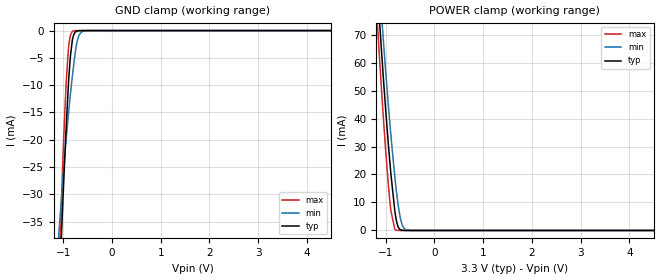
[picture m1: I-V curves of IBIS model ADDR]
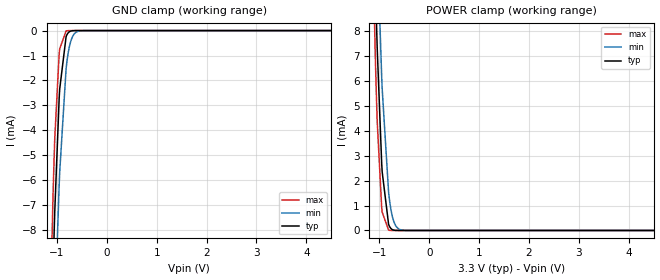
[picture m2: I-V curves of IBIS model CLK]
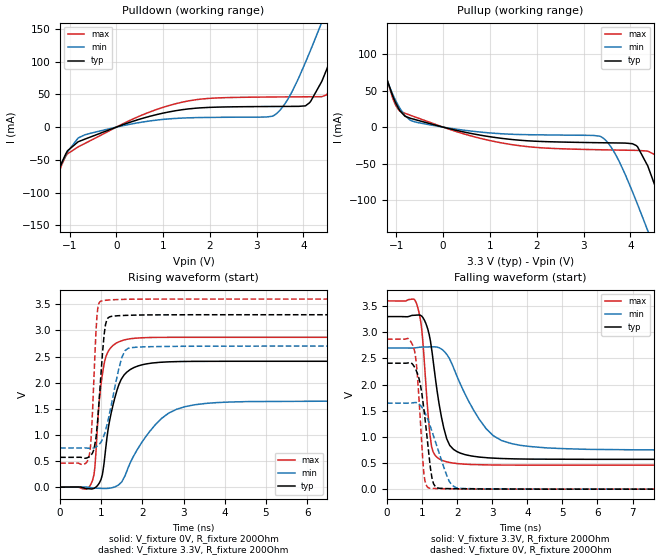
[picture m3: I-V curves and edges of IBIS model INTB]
|Texas Instruments Incorporated
| Marketing part#   Digital Voltage Range   Package-type   #pins
| FDC2114   2.7V-3.6V   QFN   16
[IBIS Ver]   4.1
[File name]   fdc2114.ibs
[File Rev]   1.0
[Date]   12/10/2014
[Source]
| Texas Instruments Incorporated.
| 12500 TI Blvd
| Dallas, TX -75243
[Notes]   Revision History:
| Rev 1.0: 12/10/2014
| - Initial version of the model
| - Model generated from simulations in TISPICE
| - C_comp although listed in numerical order of value are
|   obtained from varying PVT conditions. For PVT conditions for
|   each specific value refer the buffer description under
|   respective [Model]. IBIS model user is responsible for using
|   appropriate C_comp to simulate for Signal Integrity.
| - Warnings regarding combined Non-monotonicity of various models have been
|   reviewd and considered minor and can be ignored.
[Disclaimer]
| This model is designed as an aid for customers of Texas Instruments.
| TI and its licensors and suppliers make no warranties, either expressed
| or implied, with respect to this  model, including the warranties of
| merchantability or fitness for a particular purpose. The model is
| provided solely on an "as is" basis. The entire risk as to its quality
| and performance is with the customer.
[Copyright]
 (C) Copyright 2014 Texas Instruments Incorporated.All rights reserved.
|   Device
[Component]   FDC2114
[Manufacturer]   TI
[Package]
| QFN   16
|   typ   min   max
R_pkg   0.055   0.033   0.082
L_pkg   0.881nH   0.624nH   1.131nH
C_pkg   0.218pF   0.183pF   0.252pF
[Pin]  signal_name   model_name   R_pin   L_pin   C_pin
1   SCL   SCL   0.07306   0.978nH   0.18274pF
2   SDA   SDA   0.07559   1.01766nH   0.20668pF
3   CKIN   CLK   0.07543   1.01504nH   0.20688pF
4   ADDR   ADDR   0.08092   1.10425nH   0.19068pF
5   INTB   INTB   0.08236   1.13165nH   0.19465pF
6   SD   ADDR   0.08179   1.12348nH   0.21458pF
7   VDD   POWER   0.07866   1.06968nH   0.21147pF
8   GND   GND   0.04053   0.79295nH   0.22494pF
9   IN0A   NC   0.04363   0.92929nH   0.23597pF
10   IN0B   NC   0.03905   0.78694nH   0.25179pF
11   IN1A   NC   0.03767   0.74474nH   0.2462pF
12   IN1B   NC   0.03662   0.71322nH   0.21859pF
13   IN2A   NC   0.03341   0.62974nH   0.20896pF
14   IN2B   NC   0.03331   0.62362nH   0.23291pF
15   IN3A   NC   0.03436   0.6538nH   0.23712pF
16   IN3B   NC   0.03859   0.786nH   0.22133pF
| Models and submodels in the file (5): ADDR (Input), CLK (Input), INTB (Output), SCL (Input), SDA (I/O_open_drain)
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|   Model
[Model]   ADDR
Model_type   Input
Vinl = 0.99
Vinh = 2.31
|   typ   min   max
C_comp   0.676pF   0.666pF   0.695pF
[Voltage Range]   3.3   2.7   3.6
[Temperature Range]   27   125   -40
[Power Clamp Reference]   3.3   2.7   3.6
[GND Clamp Reference]   0   0   0
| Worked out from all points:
|   GND clamp passes 1 mA (typ) near -0.79 V on its own axis
|   POWER clamp passes 1 mA (typ) near -0.74 V on its own axis
[GND Clamp]
|   Voltage   I(typ)   I(min)   I(max)
-3.3V     -619.4mA   -393.3mA   -763.1mA
-1.092V   -49.22mA   -37.35mA   -44.76mA
-1.003V   -30.19mA   -26.61mA   -22.47mA
-943.8mV  -18.39mA   -20.21mA   -10.3mA
-894.3mV  -9.845mA   -15.28mA   -3.327mA
-854.7mV  -4.809mA   -11.73mA   -852.6uA
-815.1mV  -1.831mA   -8.493mA   -184uA
-795.3mV  -1.044mA   -6.986mA   -84.86uA
-735.9mV  -170.8uA   -2.934mA   -6.707uA
-696.3mV  -49.54uA   -1.348mA   -1.028uA
-547.8mV  -263.7nA   -41.3uA    0A
6.6V      0A         0A         0A
[POWER Clamp]
|   Voltage   I(typ)   I(min)   I(max)
-3.3V     741.9mA    707.9mA    777.5mA
-1.211V   97.25mA    108.2mA    85.62mA
-1.142V   78.32mA    90.49mA    65.34mA
-1.092V   65.31mA    78.23mA    51.56mA
-1.053V   55.31mA    68.69mA    41.1mA
-943.8mV  30.12mA    44.08mA    15.79mA
-894.3mV  20.1mA     33.88mA    6.969mA
-815.1mV  7.134mA    19.29mA    506.1uA
-785.4mV  3.858mA    14.56mA    134.6uA
-676.5mV  121.2uA    2.795mA    1.023uA
-528mV    587.8nA    67.21uA    0A
6.6V      0A         0A         0A
|   Model
[Model]   CLK
Model_type   Input
Vinl = 0.99
Vinh = 2.31
|   typ   min   max
C_comp   0.594pF   0.592pF   0.599pF
[Voltage Range]   3.3   2.7   3.6
[Temperature Range]   27   125   -40
[Power Clamp Reference]   3.3   2.7   3.6
[GND Clamp Reference]   0   0   0
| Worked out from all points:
|   GND clamp passes 1 mA (typ) near -0.86 V on its own axis
|   POWER clamp passes 1 mA (typ) near -0.86 V on its own axis
[GND Clamp]
|   Voltage   I(typ)   I(min)   I(max)
-3.3V     -281.2mA   -260.7mA   -298mA
-1.162V   -16.92mA   -20.78mA   -14.06mA
-1.082V   -10.12mA   -14.36mA   -7.027mA
-1.063V   -8.64mA    -12.89mA   -5.599mA
-1.053V   -7.94mA    -12.19mA   -4.947mA
-1.043V   -7.269mA   -11.49mA   -4.339mA
-953.7mV  -2.688mA   -6.162mA   -914.3uA
-815.1mV  -242.9uA   -1.528mA   -13.45uA
-765.6mV  -74.11uA   -807.8uA   -1.597uA
-706.2mV  -13.3uA    -337.5uA   -98.92nA
-518.1mV  -14.83nA   -7.449uA   0A
6.6V      0A         0A         0A
[POWER Clamp]
|   Voltage   I(typ)   I(min)   I(max)
-3.3V     281.2mA    260.7mA    298mA
-1.162V   16.92mA    20.78mA    14.06mA
-1.082V   10.12mA    14.36mA    7.027mA
-1.063V   8.64mA     12.89mA    5.599mA
-1.053V   7.94mA     12.19mA    4.947mA
-1.043V   7.269mA    11.49mA    4.339mA
-953.7mV  2.688mA    6.162mA    914.3uA
-815.1mV  242.9uA    1.528mA    13.45uA
-765.6mV  74.11uA    807.8uA    1.597uA
-706.2mV  13.3uA     337.5uA    99.01nA
-518.1mV  15.01nA    7.449uA    0A
6.6V      0A         0A         0A
|   Model
[Model]   INTB
Model_type   Output
Polarity   Non-Inverting
Vmeas = 1.65
Vref = 0
Cref = 1pF
Rref = 100000
|   typ   min   max
C_comp   0.767pF   0.749pF   0.775pF
[Voltage Range]   3.3   2.7   3.6
[Temperature Range]   27   125   -40
[Pullup Reference]   3.3   2.7   3.6
[Pulldown Reference]   0   0   -0
[Power Clamp Reference]   3.3   2.7   3.6
[GND Clamp Reference]   0   0   0
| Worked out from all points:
|   slope of the pulldown table from 0 to 0.495 V, typ, clamps not added: 41 ohm
|   slope of the pullup table from 0 to 0.495 V, typ, clamps not added: 67.4 ohm
|   falling waveform, V_fixture 3.3V, R_fixture 200Ohm: 20-80 % time 384ps typ, 948ps min, 215ps max; typ from 3.3 V to 0.57 V
|   rising waveform, V_fixture 0V, R_fixture 200Ohm: 20-80 % time 341ps typ, 835ps min, 192ps max; typ from 0 V to 2.41 V
|   rising waveform, V_fixture 3.3V, R_fixture 200Ohm: 20-80 % time 157ps typ, 320ps min, 106ps max; typ from 0.57 V to 3.3 V
|   falling waveform, V_fixture 0V, R_fixture 200Ohm: 20-80 % time 256ps typ, 493ps min, 169ps max; typ from 2.41 V to 0 V
[Pulldown]
|   Voltage   I(typ)   I(min)   I(max)
-3.3V     -512.1mA   -418.3mA   -599.6mA
-1.954V   -216.3mA   -182.9mA   -247.9mA
-1.439V   -106.8mA   -96.73mA   -118.3mA
-1.053V   -37.33mA   -39.04mA   -41.6mA
-676.5mV  -18.46mA   -11.86mA   -25.08mA
1.264V    25.05mA    13.32mA    35.67mA
3.363V    31.57mA    17.6mA     46.08mA
4.046V    32.73mA    99.49mA    46.38mA
4.392V    70.02mA    160.4mA    46.57mA
4.778V    144.5mA    231.2mA    94.15mA
5.036V    199.3mA    279.3mA    154mA
6.6V      547.5mA    577.4mA    558.7mA
[Pullup]
|   Voltage   I(typ)   I(min)   I(max)
-3.3V     522.3mA    449.6mA    602.8mA
-1.973V   226.4mA    199.4mA    255.9mA
-1.478V   119.9mA    110mA      130.3mA
-1.033V   35.8mA     38.79mA    32.43mA
-676.5mV  11.7mA     8.654mA    15.7mA
1.264V    -15.47mA   -9.126mA   -21.76mA
3.382V    -21.37mA   -13.43mA   -31.01mA
4.125V    -25.16mA   -101.1mA   -31.8mA
4.372V    -53.15mA   -141.8mA   -32.82mA
4.67V     -108.6mA   -192.1mA   -58.24mA
5.006V    -179.3mA   -250.2mA   -132.7mA
6.6V      -528.8mA   -530.4mA   -544.8mA
[Ramp]
R_load = 200
|   typ   min   max
dV/dt_r   1.44552/3.41029e-10   0.986914/8.35118e-10   1.72101/1.92002e-10
dV/dt_f   1.63788/3.84116e-10   1.17001/9.47826e-10   1.88487/2.146e-10
[Falling Waveform]
V_fixture = 3.3V
V_fixture_min = 2.7V
V_fixture_max = 3.6V
R_fixture = 200Ohm
C_fixture = 0F
|   Time   V(typ)   V(min)   V(max)
0s        3.3V       2.7V       3.6V
789ps     3.326V     2.701V     3.62V
961.1ps   3.321V     2.717V     3.201V
1.068ns   3.228V     2.718V     2.391V
1.312ns   2.474V     2.722V     716.9mV
1.618ns   1.169V     2.642V     539mV
1.978ns   725.1mV    2.187V     491.3mV
3.03ns    593.8mV    1.022V     461.8mV
4.549ns   573.5mV    789.1mV    458.7mV
50ns      570.2mV    750mV      458.5mV
[Rising Waveform]
V_fixture = 0V
V_fixture_min = 0V
V_fixture_max = 0V
R_fixture = 200Ohm
C_fixture = 0F
|   Time   V(typ)   V(min)   V(max)
0s        -3.948uV   -9.493uV   45.21uV
766.5ps   -35.26mV   -12.14mV   89.3mV
842.7ps   -13.61mV   -20.21mV   371.1mV
952ps     79.24mV    -23.04mV   1.659V
1.108ns   745.3mV    -26.13mV   2.486V
1.381ns   1.856V     25.11mV    2.765V
1.832ns   2.301V     661.1mV    2.851V
2.634ns   2.398V     1.416V     2.867V
4.091ns   2.409V     1.628V     2.868V
50ns      2.409V     1.645V     2.868V
[Rising Waveform]
V_fixture = 3.3V
V_fixture_min = 2.7V
V_fixture_max = 3.6V
R_fixture = 200Ohm
C_fixture = 0F
|   Time   V(typ)   V(min)   V(max)
0s        570.2mV    750mV      458.5mV
685ps     571.8mV    744.7mV    543.7mV
766.5ps   629mV      742.1mV    1.115V
868.3ps   936mV      768.2mV    2.95V
915.1ps   1.322V     793.7mV    3.43V
1.068ns   2.92V      996.1mV    3.573V
1.17ns    3.245V     1.301V     3.581V
1.497ns   3.285V     2.481V     3.593V
1.968ns   3.295V     2.683V     3.599V
50ns      3.3V       2.7V       3.6V
[Falling Waveform]
|Gnd
V_fixture = 0V
V_fixture_min = 0V
V_fixture_max = 0V
R_fixture = 200Ohm
C_fixture = 0F
|   Time   V(typ)   V(min)   V(max)
0s        2.409V     1.645V     2.868V
596.5ps   2.414V     1.644V     2.882V
766.5ps   2.353V     1.654V     2.69V
868.3ps   2.208V     1.648V     2.151V
1.048ns   1.544V     1.507V     315.8mV
1.217ns   525.8mV    1.232V     17.71mV
1.381ns   46mV       904.1mV    12.05mV
1.782ns   10.08mV    141mV      6.887mV
2.18ns    6.77mV     13.22mV    3.785mV
50ns      -4.626uV   -10.09uV   -44.14uV
